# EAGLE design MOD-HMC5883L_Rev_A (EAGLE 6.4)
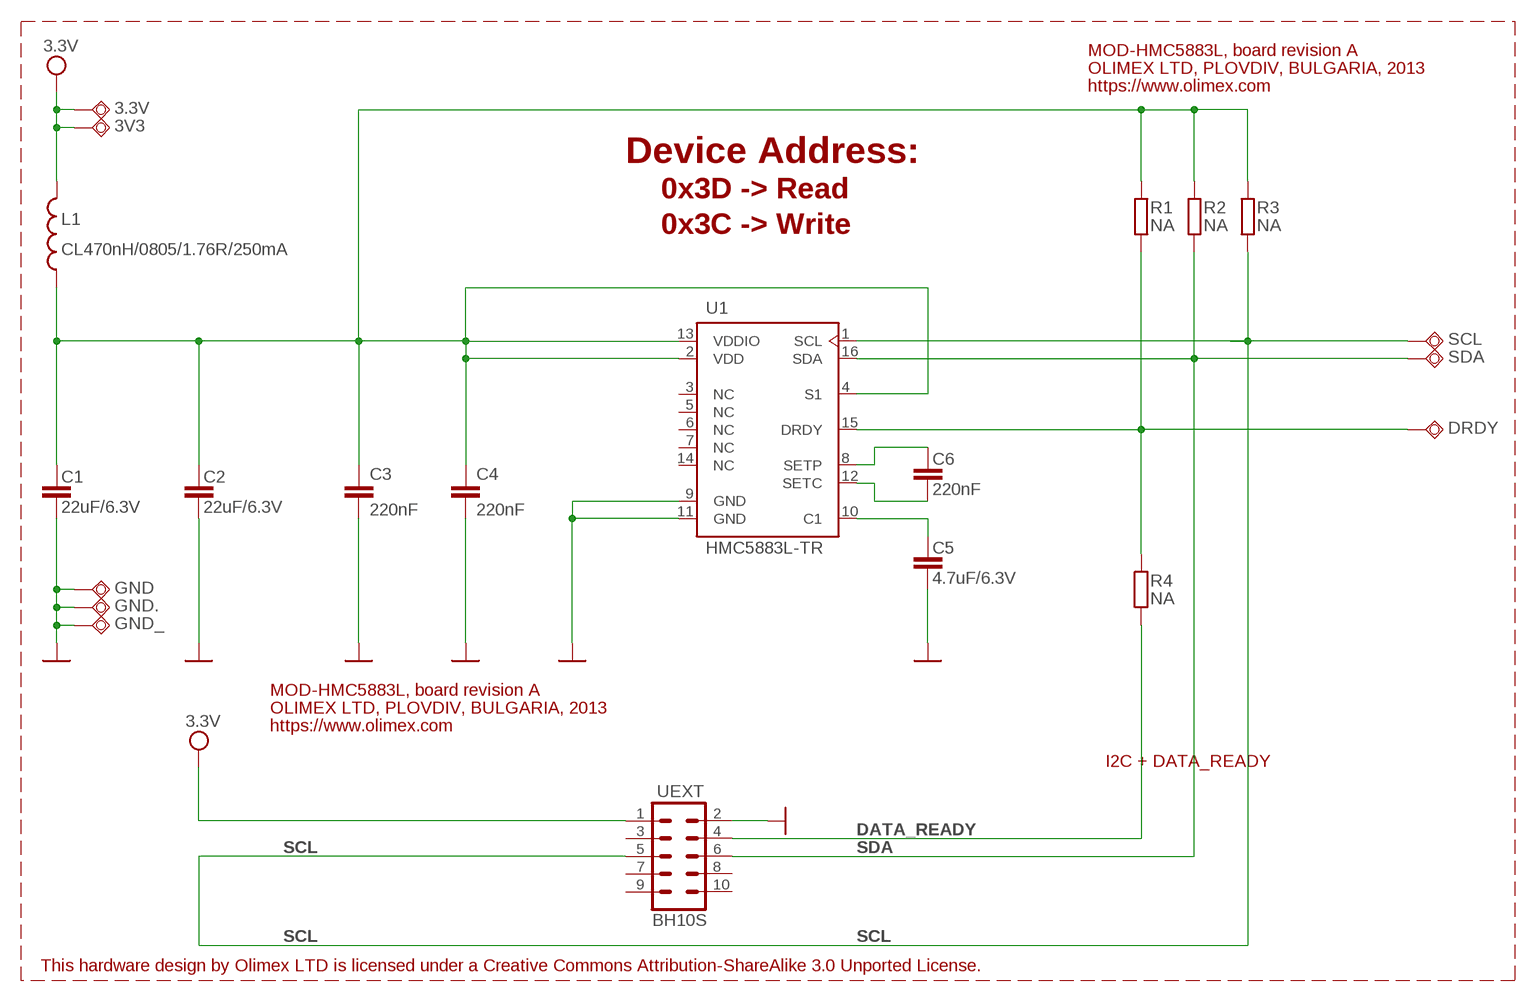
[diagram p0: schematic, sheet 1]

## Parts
3.3V  TESTPAD3  [TEST_PAD40/70/SQUARE]
3V3  TESTPAD3  [TEST_PAD40/70/SQUARE]
C1  22uF/6.3V  C-EUC0603_DWS  [C0603_DWS]
C2  22uF/6.3V  C-EUC0603_DWS  [C0603_DWS]
C3  220nF  C-EUC0603_DWS  [C0603_DWS]
C4  220nF  C-EUC0603_DWS  [C0603_DWS]
C5  4.7uF/6.3V  C-EUC0603_DWS  [C0603_DWS]
C6  220nF  C-EUC0603_DWS  [C0603_DWS]
DRDY  TESTPAD3  [TEST_PAD40/70/SQUARE]
GND  TESTPAD3  [TEST_PAD40/70/SQUARE]
GND.  TESTPAD3  [TEST_PAD40/70/SQUARE]
GND_  TESTPAD3  [TEST_PAD40/70/SQUARE]
L1  CL470nH/0805/1.76R/250mA  L-USL0805_5MIL_DWS  [L0805_5MIL_DWS]
R1  NA  R-EU_R0603_5MIL_DWS  [R0603_5MIL_DWS]
R2  NA  R-EU_R0603_5MIL_DWS  [R0603_5MIL_DWS]
R3  NA  R-EU_R0603_5MIL_DWS  [R0603_5MIL_DWS]
R4  NA  R-EU_R0603_5MIL_DWS  [R0603_5MIL_DWS]
SCL  TESTPAD3  [TEST_PAD40/70/SQUARE]
SDA  TESTPAD3  [TEST_PAD40/70/SQUARE]
U1  HMC5883L-TR  [LPCC-16]
UEXT  BH10S  ML10SMD  [ML10_PADS]

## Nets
DATA_READY: R4.2 UEXT.4
GND [PWR]: C1.2 C2.2 C3.2 C4.2 C5.2 GND..P$1(PP) GND.P$1(PP) GND_.P$1(PP) U1.9(GND) U1.11(GND) UEXT.2
N$1: C5.1 U1.10(C1)
N$2: C6.1 U1.8(SETP)
N$3: DRDY.P$1(PP) R1.2 R4.1 U1.15(DRDY)
N$4: C6.2 U1.12(SETC)
SCL: R3.2 SCL.P$1(PP) U1.1(SCL) UEXT.5
SDA: R2.2 SDA.P$1(PP) U1.16(SDA) UEXT.6
VCC: 3.3V.P$1(PP) 3V3.P$1(PP) L1.1 UEXT.1 ; supply symbol labelled 3.3V
VDD: C1.1 C2.1 C3.1 C4.1 L1.2 R1.1 R2.1 R3.1 U1.2(VDD) U1.4(S1) U1.13(VDDIO)
Unconnected: U1.3(NC) U1.5(NC) U1.6(NC) U1.7(NC) U1.14(NC) UEXT.3 UEXT.7 UEXT.8 UEXT.9 UEXT.10

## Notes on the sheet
- MOD-HMC5883L, board revision A
- OLIMEX LTD, PLOVDIV, BULGARIA, 2013
- https://www.olimex.com
- Device Address:
- 0x3D -> Read
- 0x3C -> Write
- MOD-HMC5883L, board revision A
- OLIMEX LTD, PLOVDIV, BULGARIA, 2013
- https://www.olimex.com
- I2C + DATA_READY
- This hardware design by Olimex LTD is licensed under a Creative Commons Attribution-ShareAlike 3.0 Unported License.

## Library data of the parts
3.3V 3V3 DRDY GND GND. GND_ SCL SDA = gogo:TESTPAD: drill 40mils, diameter 70mils
C1-C6 = rcl:C-EU: CAPACITOR, European symbol
L1 = rcl:L-US: INDUCTOR, American symbol
R1-R4 = rcl:R-EU_: RESISTOR, European symbol
U1 = OLIMEX_IC:HMC5883L: HMC5883L 3-Axis Digital Compass IC
UEXT = con-harting-ml:ML10: HARTING

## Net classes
0 default: width 0.203 mm, drill 0.584 mm, clearance 0.178 mm
1 PWR: width 0.203 mm, drill 0.584 mm, clearance 0.178 mm

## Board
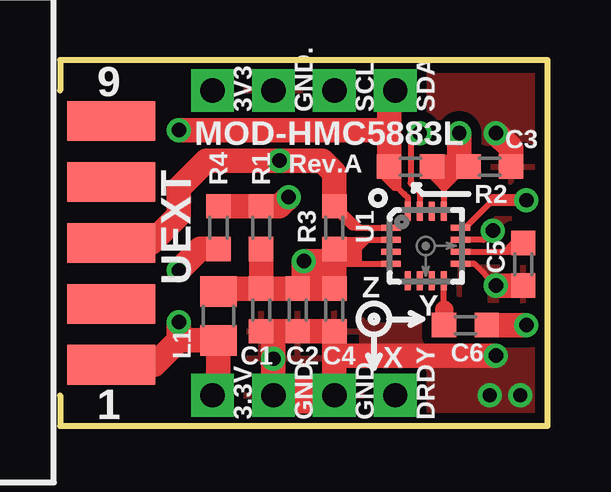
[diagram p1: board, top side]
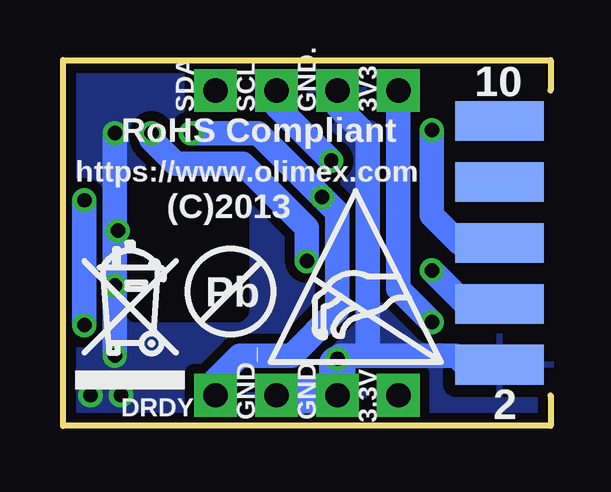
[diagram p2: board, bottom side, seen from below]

Size 20.32 x 15.24 mm. Coordinates in mm from the lower left corner, seen from the top.
Outline: 0,13.97 0,15.24 20.32,15.24 20.32,0 0,0 0,1.27
Copper layers (1+16): Top 0.035mm / dielectric 1.5mm / Bottom 0.035mm
Design rules "default": minimum track width 9.5mil, minimum drill 23mil, track to track 9.5mil, track to pad 9.5mil, pad to pad 9.5mil, via to via 10mil, smd to smd 1mil, copper to edge 10mil, drill to drill 10mil, minimum pad ring 10mil, minimum via ring 8mil, stop-mask expansion 4mil, vias tented up to drill 25mil, thermal gap 20mil
tRestrict: 4 lines
bRestrict: 4 lines

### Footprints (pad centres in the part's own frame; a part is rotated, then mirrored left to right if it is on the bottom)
TEST_PAD40/70/SQUARE = drill 1.016 pad 1.778 square: P$1 0,0
C0603_DWS = smd 1.016 x 1.016: 1 -0.889,0; 2 0.889,0
L0805_5MIL_DWS = smd 1.27 x 1.524: 1 -1.016,0; 2 1.016,0
R0603_5MIL_DWS = smd 1.016 x 1.016: 1 -0.889,0; 2 0.889,0
LPCC-16 = smd 0.8 x 0.25: 1 -1.45,0.75; 2 -1.45,0.25; 3 -1.45,-0.25; 4 -1.45,-0.75; 9 1.45,-0.75; 10 1.45,-0.25; 11 1.45,0.25; 12 1.45,0.75 | smd 0.25 x 0.8: 5 -0.75,-1.45; 6 -0.25,-1.45; 7 0.25,-1.45; 8 0.75,-1.45; 13 0.75,1.45; 14 0.25,1.45; 15 -0.25,1.45; 16 -0.75,1.45
ML10_PADS = smd 1.651 x 3.683: 1 -5.08,-0.229; 3 -2.54,-0.229; 5 0,-0.229; 7 2.54,-0.229; 9 5.08,-0.229 | smd 1.651 x 3.683 bottom: 2 -5.08,-0.229; 4 -2.54,-0.229; 6 0,-0.229; 8 2.54,-0.229; 10 5.08,-0.229

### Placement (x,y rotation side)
3.3V  6.35,1.27 90 top
3V3  6.35,13.97 90 top
C1  8.38,4.83 270 top
C2  9.91,4.83 270 top
C3  17.91,10.79 0 top
C4  11.43,4.83 270 top
C5  19.3,6.73 270 top
C6  16.89,4.19 0 top
DRDY  13.97,1.27 0 top
GND  8.89,1.27 90 top
GND.  8.89,13.97 90 top
GND_  11.43,1.27 0 top
L1  6.6,4.57 90 top
R1  8.38,8.26 90 top
R2  14.61,10.79 180 top
R3  11.43,8.26 90 top
R4  6.6,8.26 270 top
SCL  11.43,13.97 0 top
SDA  13.97,13.97 0 top
U1  15.24,7.49 0 top
U$1  [ESD_SYMBOL]  11.68,2.67 0 bottom
U$3  [PB_SMALL]  13.34,5.59 0 bottom
U$4  [RECYCLE_BIN1/8]  19.81,1.52 0 bottom
UEXT  1.91,7.62 90 top

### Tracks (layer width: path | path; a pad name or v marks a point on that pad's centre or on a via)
DATA_READY  (via drill 0.6)
  Top 1.016: v4.95,6.48 5.84,7.37 R4.2
  Bottom 0.254: UEXT.4 2.03,5.08
  Bottom 1.016: v4.95,6.48 3.56,5.08 UEXT.4
GND  (via drill 0.6)
  Top 0.254: U1.11 17.65,7.74 v18.03,8.13 | v18.16,5.84 17.26,6.74 U1.9
  Top 0.762: GND_.P$1 11.43,1.65
  Top 1.016: v18.16,5.84 C5.2 | 11.43,1.65 11.43,2.92 | 11.43,2.92 C4.2 C2.2 8.89,3.94 | 11.43,2.92 v18.16,2.92 | GND.P$1 v8.89,2.79 8.89,3.94 | 8.89,3.94 C1.2 | v18.16,12.19 18.8,11.56 C3.2
  Top 1.524: GND.P$1 GND_.P$1
  Bottom 1.016: 18.16,8.13 v18.16,5.84 v18.16,2.92 | 18.16,8.13 v18.03,8.13 | 18.16,8.13 v18.16,12.19 | 7.62,2.92 7.62,12.06 8.89,13.34 GND..P$1 | UEXT.2 3.56,2.54 3.94,2.92 7.62,2.92 | 7.62,2.92 8.76,2.92 v8.89,2.79 8.89,2.56
  Bottom 1.524: 8.89,2.56 GND.P$1 GND_.P$1
  other vias: 19.18,1.27 17.91,1.27
  pour Bottom (isolate 0.406): 0,16.51 0,-1.27 21.59,-1.27 21.59,16.51
  pour Top (isolate 0.406): 0,17.78 0,-2.54 23.75,-2.54 23.75,17.78
N$1
  Top 0.254: U1.10 18.67,7.24 18.8,7.37
  Top 0.508: 18.8,7.37 19.05,7.62 C5.1
N$2
  Top 0.254: C6.1 15.99,4.2 | U1.8 15.99,4.83 16,4.83
  Top 0.762: C6.1 16,4.83
N$3  (via drill 0.6)
  Top 0.254: U1.15 14.99,9.72 14.61,10.11 14.61,11.81 v14.99,12.19
  Top 1.016: R4.1 R1.2 9.14,9.14 v9.53,9.53
  Bottom 1.016: DRDY.P$1 13.97,1.91 12.95,2.92 10.79,2.92 8.89,4.83 8.89,8.89 v9.53,9.53 12.19,12.19 v14.99,12.19
N$4  (via drill 0.6)
  Top 0.254: U1.12 16.88,8.24 18.03,9.4
  Top 0.508: v19.43,9.4 18.03,9.4
  Top 1.016: C6.2 v19.43,4.19
  Bottom 1.016: v19.43,4.19 v19.43,9.4
SCL  (via drill 0.6)
  Top 0.254: 12.19,8.38 12.33,8.24 12.51,8.24 | 12.51,8.24 U1.1 | UEXT.5 1.91,7.62 | 12.51,8.24 12.37,8.38
  Top 0.508: R3.2 12.19,8.38
  Top 1.016: R3.2 11.43,10.54 10.92,11.05 v9.14,11.05 6.1,11.05 4.95,9.91 4.95,8.76 3.81,7.62 UEXT.5
  Bottom 1.016: v9.14,11.05 11.43,13.34 SCL.P$1
SDA  (via drill 0.6)
  Top 0.254: U1.16 14.49,9.51 14.35,9.65 13.97,10.03
  Top 0.508: R2.2 13.97,10.79 13.97,10.03 13.46,10.54 13.46,10.92
  Top 1.016: 13.72,12.32 R2.2 | 13.72,12.32 13.72,13.72 SDA.P$1 | v4.95,12.32 13.72,12.32
  Bottom 1.016: v4.95,12.32 4.95,8.76 3.81,7.62 UEXT.6
VCC  (via drill 0.6)
  Top 1.016: 3.3V.P$1 6.22,1.27 6.6,1.65 L1.1 4.95,3.56 | 4.95,3.56 v4.95,4.32 | UEXT.1 3.94,2.54 4.95,3.56
  Bottom 1.016: 3V3.P$1 6.35,5.71 v4.95,4.32
VDD  (via drill 0.6)
  Top 0.254: U1.2 11.81,7.74 11.61,7.54 | 11.61,7.54 R3.1 12.06,7.37 12.06,6.86 12.19,6.86 12.19,7.37 12.32,7.37 12.32,6.86 12.45,6.86 12.45,7.37 12.62,7.54 | 12.62,7.54 12.8,7.72 | 11.43,6.74 U1.4 | 16,10.03 15.99,10.03 U1.13 | 11.61,7.54 12.62,7.54
  Top 0.508: 16,10.79 16,10.03 | 16.76,10.79 16,10.03 | 16,10.03 15.24,10.79
  Top 1.016: L1.2 6.48,5.71 C1.1 | 10.16,5.71 C2.1 C1.1 | 10.16,5.71 10.79,5.71 | 10.79,5.71 C4.1 11.43,6.74 11.43,6.86 | v16.64,12.19 16.64,10.79 | 10.79,6.86 11.43,6.86 | 10.79,6.86 v10.16,6.86 10.16,5.71 | R2.1 16,10.79 16.64,10.79 | 16.64,10.79 16.76,10.79 C3.1 | C1.1 R1.1 | 11.43,6.86 R3.1 | 10.79,5.71 10.79,6.86
  Bottom 1.016: v10.16,6.86 10.16,8.26 12.83,10.92 15.62,10.92 16.64,11.94 v16.64,12.19

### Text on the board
tNames: MOD-HMC5883L | Rev.A | Z | Y | X
bNames: RoHS Compliant | https://www.olimex.com | (C)2013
